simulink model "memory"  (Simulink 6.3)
settings: Solver=ode45  StartTime=0.0  StopTime=25.0  RelTol=1e-3
undefined symbols (not defined in the file or in its folder): netlist
libraries: xbsIndex_r4 x19, adlibrary2 x2

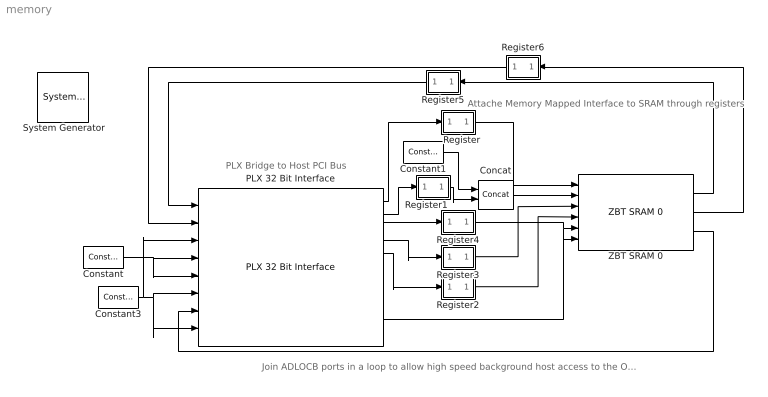
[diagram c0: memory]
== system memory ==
  note: PLX Bridge to Host PCI Bus
  note: Attache Memory Mapped Interface to SRAM through registers
  note: Join ADLOCB ports in a loop to allow high speed background host access to the Off Chip Ram
  " System Generator" : xbsIndex_r4/ System Generator  Tag=genX  xilinxfamily=Virtex4  part=xc4vsx55  speed=-10  package=ff1148  synthesis_tool=XST  directory=./netlist  testbench=off  simulink_period=1  sysclk_period=6  incr_netlist=off  trim_vbits=Everywhere in SubSystem  dbl_ovrd=According to Block Masks  core_generation=According to Block Masks  run_coregen=off  deprecated_control=off  eval_field=0  block_type=sysgen
  Concat : xbsIndex_r4/Concat  num_inputs=2  dbl_ovrd=off  block_type=concat
  Constant : xbsIndex_r4/Constant  arith_type=Boolean  const=0  n_bits=1  bin_pt=0  explicit_period=on  period=1  equ=P=C  opselect=C  inp2=PCIN>>17  opr=+  inp1=P  carry=CIN  dbl_ovrd=off  block_type=constant
  Constant1 : xbsIndex_r4/Constant  arith_type=Unsigned  const=0  n_bits=5  bin_pt=0  explicit_period=on  period=1  equ=P=C  opselect=C  inp2=PCIN>>17  opr=+  inp1=P  carry=CIN  dbl_ovrd=off  block_type=constant
  Constant3 : xbsIndex_r4/Constant  arith_type=Unsigned  const=0  n_bits=32  bin_pt=0  explicit_period=on  period=1  equ=P=C  opselect=C  inp2=PCIN>>17  opr=+  inp1=P  carry=CIN  dbl_ovrd=off  block_type=constant
  PLX 32 Bit Interface : adlibrary2/ADM-XRC-II/PLX 32 Bit Interface  program='slave_write 0x0000 0xabcd1234;slave_read 0x0000'  clock_ratio=1.5
  Register : Subsystem
  Register1 : Subsystem
  Register2 : Subsystem
  Register3 : Subsystem
  Register4 : Subsystem
  Register5 : Subsystem  Orientation=left
  Register6 : Subsystem  Orientation=left
  ZBT SRAM 0 : adlibrary2/ADM-XRC-4LX//SX/ZBT SRAM 0
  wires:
  Constant/1 -> PLX 32 Bit Interface/4, PLX 32 Bit Interface/5
  Constant3/1 -> PLX 32 Bit Interface/3, PLX 32 Bit Interface/6, PLX 32 Bit Interface/8
  PLX 32 Bit Interface/3 -> Register4/1(in0)
  PLX 32 Bit Interface/5 -> Register2/1(in0)
  PLX 32 Bit Interface/4 -> Register3/1(in0)
  PLX 32 Bit Interface/2 -> Register1/1(in0)
  PLX 32 Bit Interface/1 -> Register/1(in0)
  PLX 32 Bit Interface/10 -> ZBT SRAM 0/6
  ZBT SRAM 0/3 -> PLX 32 Bit Interface/7
  ZBT SRAM 0/2 -> Register6/1(in0)
  ZBT SRAM 0/1 -> Register5/1(in0)
  Register/1(out0) -> ZBT SRAM 0/1
  Register2/1(out0) -> ZBT SRAM 0/4
  Register3/1(out0) -> ZBT SRAM 0/3
  Register4/1(out0) -> ZBT SRAM 0/5
  Concat/1 -> ZBT SRAM 0/2
  Constant1/1 -> Concat/1
  Register1/1(out0) -> Concat/2
  Register5/1(out0) -> PLX 32 Bit Interface/1
  Register6/1(out0) -> PLX 32 Bit Interface/2

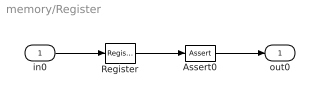
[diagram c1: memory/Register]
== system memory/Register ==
  in0 : Inport
  Assert0 : xbsIndex_r4/Assert  assert_type=off  type_source=Explicitly  arith_type="Signed  (2's comp)"  n_bits=16  bin_pt=14  assert_rate=on  rate_source=Explicitly  period=1  output_port=on  block_type=assert
  Register : xbsIndex_r4/Register  init=0  rst=off  en=off  dbl_ovrd=off  block_type=register
  out0 : Outport
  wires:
  in0/1 -> Register/1
  Register/1 -> Assert0/1
  Assert0/1 -> out0/1

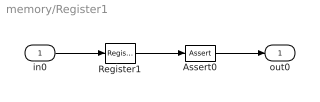
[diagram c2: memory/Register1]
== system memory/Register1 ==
  in0 : Inport
  Assert0 : xbsIndex_r4/Assert  assert_type=off  type_source=Explicitly  arith_type="Signed  (2's comp)"  n_bits=16  bin_pt=14  assert_rate=on  rate_source=Explicitly  period=1  output_port=on  block_type=assert
  Register1 : xbsIndex_r4/Register  init=0  rst=off  en=off  dbl_ovrd=off  block_type=register
  out0 : Outport
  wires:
  in0/1 -> Register1/1
  Register1/1 -> Assert0/1
  Assert0/1 -> out0/1

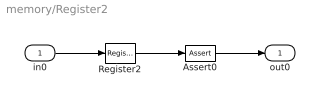
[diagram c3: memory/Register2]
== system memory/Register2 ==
  in0 : Inport
  Assert0 : xbsIndex_r4/Assert  assert_type=off  type_source=Explicitly  arith_type="Signed  (2's comp)"  n_bits=16  bin_pt=14  assert_rate=on  rate_source=Explicitly  period=1  output_port=on  block_type=assert
  Register2 : xbsIndex_r4/Register  init=0  rst=off  en=off  dbl_ovrd=off  block_type=register
  out0 : Outport
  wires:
  in0/1 -> Register2/1
  Register2/1 -> Assert0/1
  Assert0/1 -> out0/1

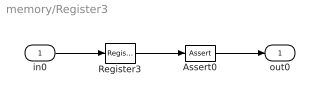
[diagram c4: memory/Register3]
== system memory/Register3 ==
  in0 : Inport
  Assert0 : xbsIndex_r4/Assert  assert_type=off  type_source=Explicitly  arith_type="Signed  (2's comp)"  n_bits=16  bin_pt=14  assert_rate=on  rate_source=Explicitly  period=1  output_port=on  block_type=assert
  Register3 : xbsIndex_r4/Register  init=0  rst=off  en=off  dbl_ovrd=off  block_type=register
  out0 : Outport
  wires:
  in0/1 -> Register3/1
  Register3/1 -> Assert0/1
  Assert0/1 -> out0/1

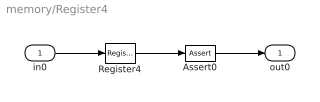
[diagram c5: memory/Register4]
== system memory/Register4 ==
  in0 : Inport
  Assert0 : xbsIndex_r4/Assert  assert_type=off  type_source=Explicitly  arith_type="Signed  (2's comp)"  n_bits=16  bin_pt=14  assert_rate=on  rate_source=Explicitly  period=1  output_port=on  block_type=assert
  Register4 : xbsIndex_r4/Register  init=0  rst=off  en=off  dbl_ovrd=off  block_type=register
  out0 : Outport
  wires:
  in0/1 -> Register4/1
  Register4/1 -> Assert0/1
  Assert0/1 -> out0/1

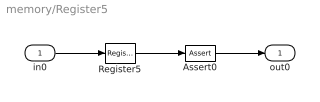
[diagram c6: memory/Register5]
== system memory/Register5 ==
  in0 : Inport
  Assert0 : xbsIndex_r4/Assert  assert_type=off  type_source=Explicitly  arith_type="Signed  (2's comp)"  n_bits=16  bin_pt=14  assert_rate=on  rate_source=Explicitly  period=1  output_port=on  block_type=assert
  Register5 : xbsIndex_r4/Register  init=0  rst=off  en=off  dbl_ovrd=off  block_type=register
  out0 : Outport
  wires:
  in0/1 -> Register5/1
  Register5/1 -> Assert0/1
  Assert0/1 -> out0/1

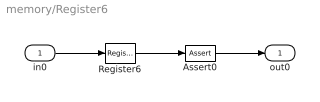
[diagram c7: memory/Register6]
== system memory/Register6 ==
  in0 : Inport
  Assert0 : xbsIndex_r4/Assert  assert_type=off  type_source=Explicitly  arith_type="Signed  (2's comp)"  n_bits=16  bin_pt=14  assert_rate=on  rate_source=Explicitly  period=1  output_port=on  block_type=assert
  Register6 : xbsIndex_r4/Register  init=0  rst=off  en=off  dbl_ovrd=off  block_type=register
  out0 : Outport
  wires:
  in0/1 -> Register6/1
  Register6/1 -> Assert0/1
  Assert0/1 -> out0/1
